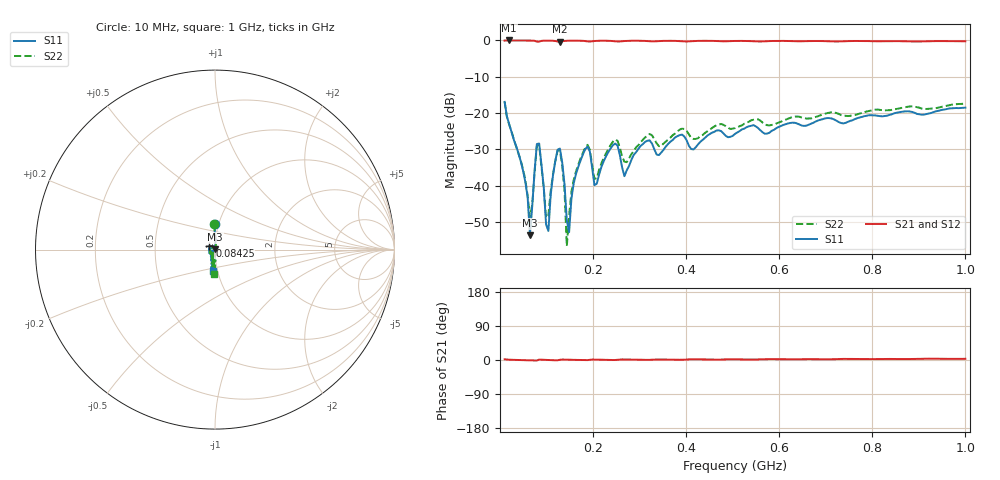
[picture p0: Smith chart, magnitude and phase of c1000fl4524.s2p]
!Agilent Technologies,N5234A,MY52241123,A.10.00.00
!Agilent N5234A: A.10.00.00
!Date: Monday, January 21, 2019 13:55:52
!Correction: S11(Full 2 Port(1,2))
!S21(Full 2 Port(1,2))
!S12(Full 2 Port(1,2))
!S22(Full 2 Port(1,2))
!S2P File: Measurements: S11, S21, S12, S22:
# Hz S  dB  R 50
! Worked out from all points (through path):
!   201 points, 10 MHz to 1 GHz, reference 50 ohm
!   highest |S21| = -0.02 dB at 19.9 MHz (marker M1); lowest = -0.4 dB at 128.8 MHz (marker M2)
!   lowest |S11| = -53.7 dB at 64.45 MHz (marker M3), VSWR 1.00, Z = 50.1 + j0.144 ohm
!   |S11| at or under -10 dB: start of sweep to end of sweep
!   |S22| runs from -56.6 to -16.9 dB; largest |S21 - S12| = 0.0027
!   S11 on the Smith chart (normalised r, x): 10 MHz: 0.96, +0.28; 84.25 MHz: 0.94, +0.04; 1 GHz: 0.95, -0.23
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1e7  -16.92 90.8  -0.04 1.8  -0.04 1.8  -16.85 92.0
1.99e7  -23.08 89.3  -0.02 0.7  -0.01 0.7  -23.21 88.5
5.455e7  -39.00 77.4  -0.03 -0.2  -0.02 -0.2  -38.45 69.9
6.445e7  -53.67 43.7  -0.04 -0.5  -0.03 -0.5  -48.63 25.9
7.93e7  -28.53 -148.4  -0.33 -1.4  -0.33 -1.5  -29.00 -145.1
8.425e7  -28.38 145.0  -0.33 1.1  -0.33 1.1  -28.84 144.5
1.0405e8  -52.47 -105.8  -0.07 0.0  -0.07 -0.0  -48.21 -43.8
1.1395e8  -37.17 -110.5  -0.10 -0.5  -0.10 -0.5  -36.89 -92.0
1.288e8  -29.76 174.6  -0.37 0.6  -0.36 0.6  -30.34 -175.9
1.387e8  -39.57 127.8  -0.14 1.2  -0.14 1.1  -41.25 129.7
1.4365e8  -49.57 124.8  -0.10 0.9  -0.10 0.9  -56.65 94.3
1.486e8  -52.81 -88.9  -0.08 0.7  -0.08 0.7  -48.25 -52.2
1.5355e8  -43.54 -81.4  -0.07 0.5  -0.07 0.5  -41.67 -62.4
1.783e8  -31.38 -104.0  -0.12 -0.3  -0.12 -0.3  -30.93 -89.7
2.0305e8  -39.86 -146.5  -0.17 1.2  -0.17 1.2  -38.11 -129.0
2.476e8  -28.40 -122.0  -0.25 0.0  -0.25 -0.0  -27.31 -106.1
2.674e8  -37.38 -124.6  -0.17 1.5  -0.17 1.5  -33.40 -110.8
3.4165e8  -31.56 -108.6  -0.17 1.5  -0.18 1.5  -29.11 -102.0
5.05e8  -25.73 -94.3  -0.15 1.8  -0.16 1.8  -24.16 -92.1
6.733e8  -22.68 -94.5  -0.17 2.2  -0.18 2.3  -21.33 -92.2
8.3665e8  -20.51 -94.8  -0.21 2.8  -0.21 2.8  -19.22 -93.2
1e9  -18.51 -95.8  -0.24 3.1  -0.24 3.1  -17.38 -92.2
